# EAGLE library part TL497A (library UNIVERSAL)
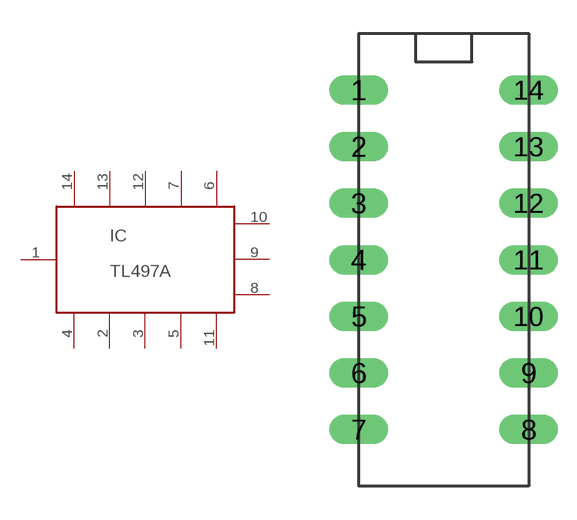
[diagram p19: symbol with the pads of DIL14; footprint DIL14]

Designator prefix IC

## TL497A  [DIL14]
1  1
2  2
3  3
4  4
5  5
6  6
7  7
8  8
9  9
10  10
11  11
12  12
13  13
14  14

## Footprint DIL14 (pad centres in mm)
drill 0.813 pad 1.092 long: 1 0,0; 2 0,-2.54; 3 0,-5.08; 4 0,-7.62; 5 0,-10.16; 6 0,-12.7; 7 0,-15.24; 8 7.62,-15.24; 9 7.62,-12.7; 10 7.62,-10.16; 11 7.62,-7.62; 12 7.62,-5.08; 13 7.62,-2.54; 14 7.62,0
